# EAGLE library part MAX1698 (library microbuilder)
MX1698/MAX1698A - Step-Up Current Regulator for LEDs Digikey: MAX1698EUB+-ND
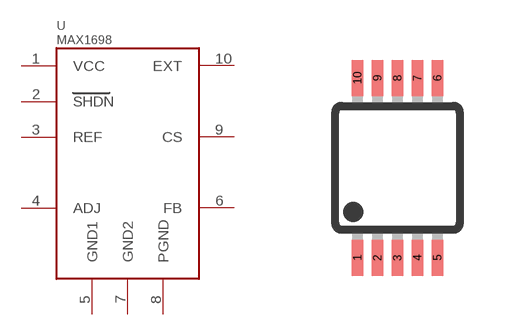
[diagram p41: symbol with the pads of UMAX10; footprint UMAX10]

Designator prefix U

## MAX1698  [UMAX10]
1  VCC
2  SHDN
3  REF
4  ADJ
5  GND1
6  FB
7  GND2
8  PGND
9  CS
10  EXT

## Footprint UMAX10 (pad centres in mm)
micro MAX Package
smd 0.29 x 0.9: 1 -1,-2.25; 2 -0.5,-2.25; 3 0,-2.25; 4 0.5,-2.25; 5 1,-2.25; 6 1,2.25; 7 0.5,2.25; 8 0,2.25; 9 -0.5,2.25; 10 -1,2.25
